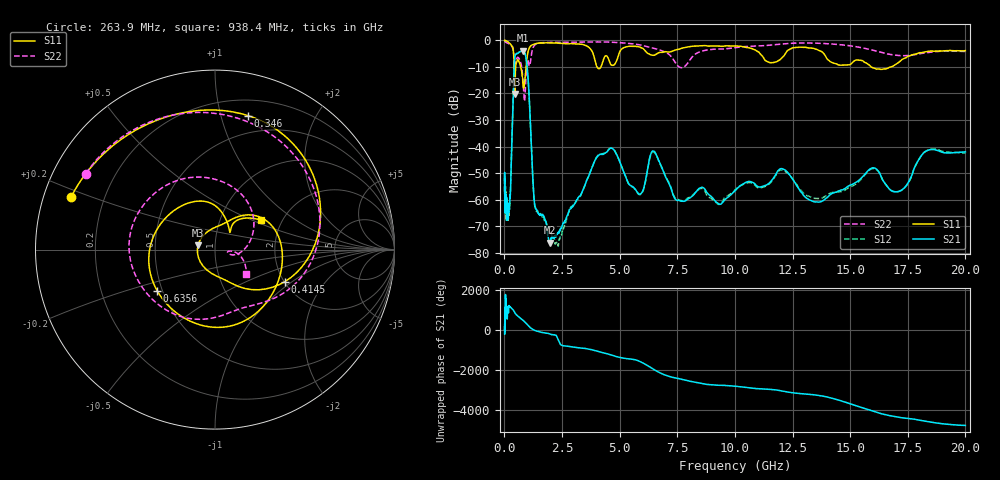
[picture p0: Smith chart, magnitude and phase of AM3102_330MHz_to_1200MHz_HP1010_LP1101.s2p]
! Date/Time: Tue, Sep 11, 2018 5:19 PM
! Network Analyzer: Agilent Technologies E8362B Rev: A.07.50.63
! Sweep from 0.010 to 20.000 GHz, 1601 Points, Sweep Type: LOG
! Power Supply: 4.949 V, 0.001 A
# Hz S DB R 50
!freq MagS11 AngS11 MagS21 AngS21 MagS12 AngS12 MagS22 AngS22
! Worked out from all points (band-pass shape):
!   1601 points, 10 MHz to 20 GHz, reference 50 ohm
!   highest |S21| = -3.85 dB at 798.4 MHz (marker M1); lowest = -76.1 dB at 1.988 GHz (marker M2)
!   |S21| within 3 dB of the highest: 443.9 MHz to 945 MHz (501.1 MHz wide, 72.2 % of centre)
!   lowest |S11| = -20.2 dB at 451.5 MHz (marker M3), VSWR 1.22, Z = 41.3 + j2.09 ohm
!   |S11| at or under -10 dB: 706.1 MHz to 942.3 MHz (236.2 MHz wide, 28.7 % of centre); 4.017 GHz to 4.188 GHz (171.1 MHz wide, 4.17 % of centre); 15.91 GHz to 16.77 GHz (853.5 MHz wide, 5.22 % of centre)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
!   |S22| runs from -22.9 to -0.2 dB; largest |S21 - S12| = 0.0098
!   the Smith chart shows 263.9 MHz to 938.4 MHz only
!   S11 on the Smith chart (normalised r, x): 263.9 MHz: 0.08, +0.18; 346 MHz: 0.33, +1.22; 414.5 MHz: 2.02, -0.88; 635.6 MHz: 0.47, -0.25; 938.4 MHz: 1.56, +0.57
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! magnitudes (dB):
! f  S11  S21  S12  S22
! 10 MHz  0.0  -57.7  -53.2  -0.2
! 35.55 MHz  0.0  -62.1  -63.9  -0.5
! 126.4 MHz  -0.4  -65.6  -61.1  -1.0
! 263.9 MHz  -1.4  -56.5  -56.0  -1.6
! 346 MHz  -2.3  -31.5  -31.6  -2.6
! 414.5 MHz  -7.4  -11.4  -11.4  -5.9
! 447.2 MHz  -20.0  -6.6  -6.6  -8.7
! 451.5 MHz  -20.2  -6.3  -6.4  -8.9
! 635.6 MHz  -8.1  -4.4  -4.5  -6.8
! 798.4 MHz  -15.9  -3.9  -3.9  -14.1
! 938.4 MHz  -10.4  -6.5  -6.6  -13.1
! 1.302 GHz  -1.4  -60.9  -61.3  -1.9
! 1.59 GHz  -1.0  -65.5  -65.7  -0.9
! 1.988 GHz  -0.9  -76.1  -72.5  -0.8
! 2.392 GHz  -1.1  -71.6  -74.9  -0.7
! 4.543 GHz  -7.5  -41.0  -40.8  -0.6
! 5.652 GHz  -2.2  -55.8  -55.9  -1.4
! 6.518 GHz  -5.6  -41.9  -42.3  -3.0
! 7.625 GHz  -3.2  -60.5  -60.2  -10.2
! 12.03 GHz  -6.6  -48.3  -48.8  -1.4
! 13.61 GHz  -3.7  -60.9  -59.5  -1.1
! 20 GHz  -3.9  -42.0  -42.5  -4.2
